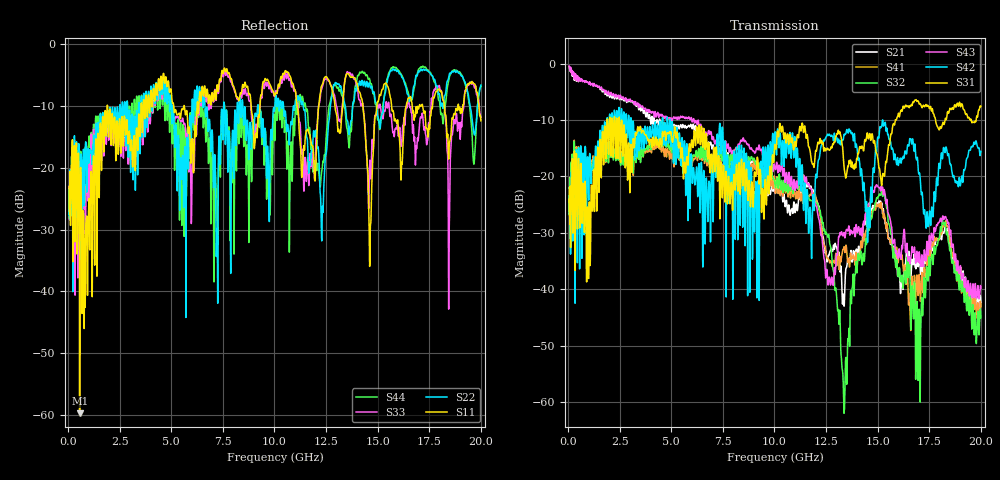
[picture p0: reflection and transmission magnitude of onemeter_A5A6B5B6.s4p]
! FILE: D:\iPass\iPassCable1005\iPassCable\SOLT_cal\onemeter_A5A6B5B6.s4p
# MHz S MA R 50.00
! FREQ  S11  S12  S13  S14
!  S21  S22  S23  S24
!  S31  S32  S33  S34
!  S41  S42  S43  S44
!  MAG  ANG  MAG  ANG  MAG  ANG  MAG  ANG
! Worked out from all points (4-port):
!   1996 points, 50 MHz to 20 GHz, reference 50 ohm
!   strongest paths, dB at 50 MHz, 5.04 GHz, 10.03 GHz, 15.02 GHz, 20 GHz:
!     S31: -24.0, -13.7, -14.4, -17.1, -7.6
!     S42: -24.8, -10.3, -12.1, -13.0, -15.6
!     S43: -0.4, -10.1, -18.7, -21.9, -39.9
!     S32: -26.6, -14.6, -21.6, -23.6, -45.1
!     S41: -26.5, -16.2, -22.1, -25.3, -43.1
!     S21: -0.5, -11.0, -22.7, -24.8, -42.4
!   lowest |S11| = -59.7 dB at 560 MHz (marker M1), VSWR 1.00, Z = 50.1 + j0.0238 ohm
!   |S11| at or under -10 dB: start of sweep to 1.897 GHz; 1.91 GHz to 3.535 GHz (1.625 GHz wide, 59.7 % of centre); 11.1 GHz to 12.14 GHz (1.039 GHz wide, 8.94 % of centre)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
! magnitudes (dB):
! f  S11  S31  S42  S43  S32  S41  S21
! 50 MHz  -23.0  -24.0  -24.8  -0.4  -26.6  -26.5  -0.5
! 560 MHz  -59.7  -27.9  -36.4  -2.6  -18.5  -18.3  -2.7
! 11.26 GHz  -16.6  -11.6  -19.7  -20.7  -22.3  -24.3  -23.0
! 13.35 GHz  -7.7  -17.4  -13.1  -30.2  -59.7  -32.8  -41.5
! 14.63 GHz  -32.2  -12.6  -27.7  -25.0  -28.1  -28.0  -25.3
! 15.13 GHz  -8.3  -19.9  -11.3  -22.6  -23.3  -25.6  -24.4
! 20 GHz  -12.4  -7.6  -15.6  -39.9  -45.1  -43.1  -42.4
